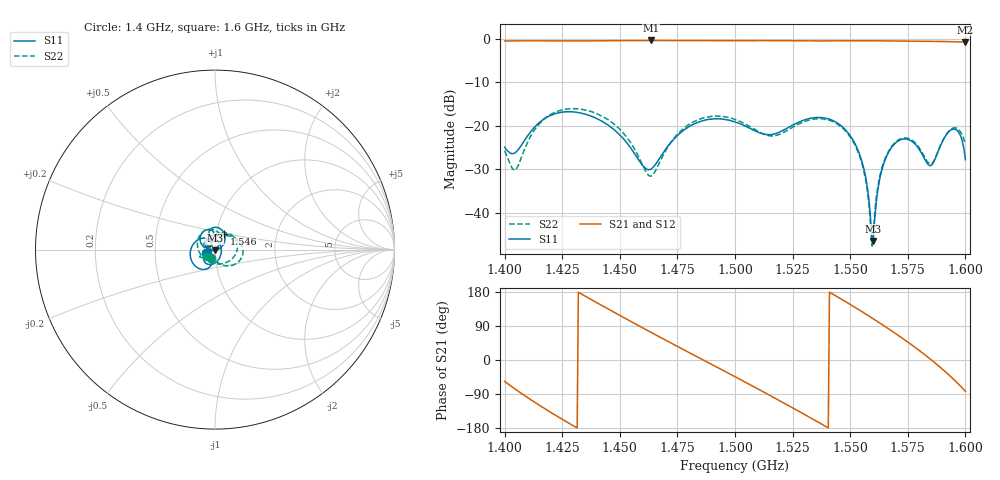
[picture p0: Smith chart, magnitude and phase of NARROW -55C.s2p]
!Agilent Technologies,E8364B,MY43040699,A.07.50.67
!Agilent E8364B: A.07.50.67
!Date: Wednesday, June 25, 2025 05:52:56
!Correction: S11(Full 2 Port(1,2))
!S21(Full 2 Port(1,2))
!S12(Full 2 Port(1,2))
!S22(Full 2 Port(1,2))
!S2P File: Measurements: S11, S21, S12, S22:
# Hz S  dB  R 50
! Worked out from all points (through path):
!   401 points, 1.4 GHz to 1.6 GHz, reference 50 ohm
!   highest |S21| = -0.40 dB at 1.464 GHz (marker M1); lowest = -0.8 dB at 1.6 GHz (marker M2)
!   lowest |S11| = -46.5 dB at 1.56 GHz (marker M3), VSWR 1.01, Z = 49.9 - j0.458 ohm
!   |S11| at or under -10 dB: start of sweep to end of sweep
!   |S22| runs from -47.7 to -16.1 dB; largest |S21 - S12| = 0.0012
!   S11 on the Smith chart (normalised r, x): 1.4 GHz: 0.90, -0.04; 1.546 GHz: 1.09, +0.19; 1.6 GHz: 0.92, -0.02
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1.4e9  -24.96 -158.5  -0.52 -56.5  -0.52 -56.5  -25.76 -114.5
1.405e9  -26.03 -122.0  -0.49 -78.5  -0.49 -78.5  -30.03 150.8
1.414e9  -19.78 -107.3  -0.50 -115.2  -0.50 -115.2  -20.23 52.6
1.424e9  -16.99 -136.6  -0.53 -152.8  -0.52 -152.8  -16.50 11.2
1.4335e9  -17.13 -172.7  -0.52 173.6  -0.51 173.6  -16.24 -18.2
1.4495e9  -21.86 128.3  -0.44 119.3  -0.44 119.3  -20.57 -65.2
1.4635e9  -30.00 147.8  -0.40 73.1  -0.40 73.1  -31.57 -176.6
1.467e9  -27.69 163.9  -0.41 61.7  -0.40 61.7  -28.74 133.3
1.4835e9  -19.29 139.1  -0.46 8.6  -0.45 8.6  -18.71 52.1
1.5e9  -19.13 100.6  -0.46 -44.0  -0.46 -44.0  -18.55 -11.4
1.5165e9  -21.98 104.8  -0.44 -97.9  -0.44 -97.9  -22.35 -120.8
1.5335e9  -18.22 95.2  -0.50 -155.0  -0.49 -155.0  -18.54 130.2
1.546e9  -19.97 58.7  -0.49 161.2  -0.49 161.2  -20.22 79.5
1.5545e9  -27.24 25.3  -0.46 129.9  -0.46 129.9  -27.62 50.8
1.559e9  -42.54 -22.1  -0.47 112.6  -0.47 112.6  -44.33 71.9
1.56e9  -46.46 -105.2  -0.47 108.7  -0.47 108.7  -45.10 155.7
1.563e9  -31.77 -173.4  -0.48 96.9  -0.48 96.9  -31.27 -175.1
1.567e9  -25.78 164.2  -0.50 80.8  -0.50 80.8  -25.54 174.9
1.5755e9  -23.23 118.3  -0.54 45.1  -0.54 45.1  -22.97 150.2
1.585e9  -29.14 2.4  -0.57 1.4  -0.57 1.4  -28.84 177.9
1.5945e9  -20.80 -118.4  -0.69 -48.7  -0.69 -48.7  -20.58 -152.8
1.6e9  -27.80 -164.1  -0.77 -82.6  -0.77 -82.6  -24.12 -144.2
